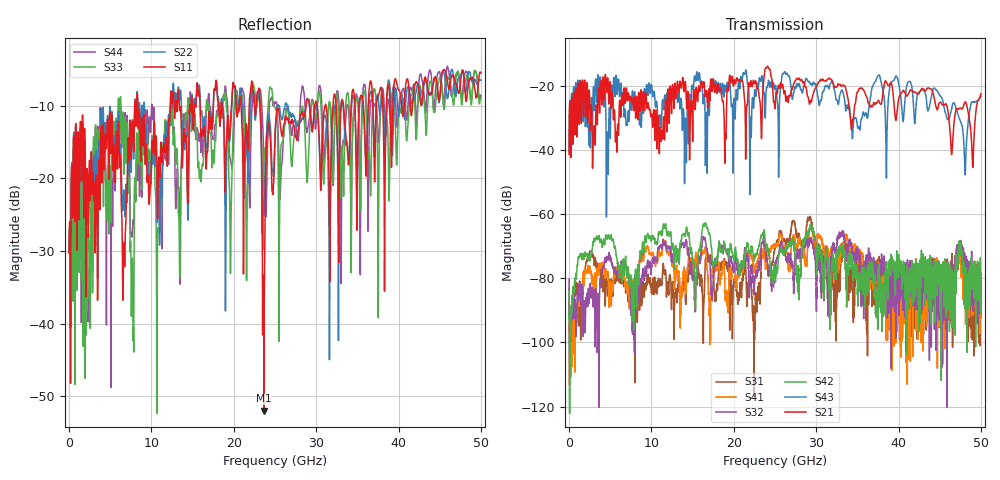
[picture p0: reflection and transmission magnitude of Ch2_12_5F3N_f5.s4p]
!Agilent Technologies,N5247A,US51170199,A.09.90.13
!Agilent N5247A: A.09.90.13
!Date: Tuesday, December 08, 2015 12:27:27
!Correction: S11(Full 4 Port(1,2,3,4))
!S12(Full 4 Port(1,2,3,4))
!S13(Full 4 Port(1,2,3,4))
!S14(Full 4 Port(1,2,3,4))
!S21(Full 4 Port(1,2,3,4))
!S22(Full 4 Port(1,2,3,4))
!S23(Full 4 Port(1,2,3,4))
!S24(Full 4 Port(1,2,3,4))
!S31(Full 4 Port(1,2,3,4))
!S32(Full 4 Port(1,2,3,4))
!S33(Full 4 Port(1,2,3,4))
!S34(Full 4 Port(1,2,3,4))
!S41(Full 4 Port(1,2,3,4))
!S42(Full 4 Port(1,2,3,4))
!S43(Full 4 Port(1,2,3,4))
!S44(Full 4 Port(1,2,3,4))
!S4P File: Measurements: <S11,S12,S13,S14>,
!<S21,S22,S23,S24>,
!<S31,S32,S33,S34>,
!<S41,S42,S43,S44>:
# Hz S  dB  R 50
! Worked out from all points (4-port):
!   3201 points, 10 MHz to 50 GHz, reference 50 ohm
!   strongest paths, dB at 10 MHz, 12.51 GHz, 25 GHz, 37.5 GHz, 50 GHz:
!     S21: -41.3, -21.8, -27.1, -24.6, -22.4
!     S43: -40.5, -22.4, -20.6, -16.9, -23.3
!     S42: -83.8, -71.1, -79.6, -80.6, -82.1
!     S32: -80.2, -72.6, -76.5, -78.3, -82.8
!     S41: -94.4, -75.5, -69.5, -78.8, -83.7
!     S31: -83.1, -83.8, -70.7, -74.2, -92.4
!   lowest |S11| = -52.0 dB at 23.66 GHz (marker M1), VSWR 1.01, Z = 50.2 - j0.104 ohm
!   |S11| at or under -10 dB: start of sweep to 7.975 GHz; 8.341 GHz to 12.29 GHz (3.949 GHz wide, 38.3 % of centre); 23.21 GHz to 28.79 GHz (5.586 GHz wide, 21.5 % of centre)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
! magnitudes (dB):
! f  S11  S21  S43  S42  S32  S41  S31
! 10 MHz  -30.2  -41.3  -40.5  -83.8  -80.2  -94.4  -83.1
! 22.19 GHz  -6.6  -19.9  -26.8  -70.0  -76.7  -73.0  -86.3
! 23.66 GHz  -52.0  -17.7  -22.0  -64.9  -66.2  -70.7  -69.3
! 25.35 GHz  -10.3  -20.8  -26.7  -77.0  -74.3  -69.2  -68.4
! 39.71 GHz  -6.6  -30.6  -16.9  -80.2  -82.4  -88.1  -82.6
! 48.09 GHz  -8.1  -25.0  -47.7  -89.5  -75.5  -80.1  -78.2
! 50 GHz  -5.4  -22.4  -23.3  -82.1  -82.8  -83.7  -92.4
